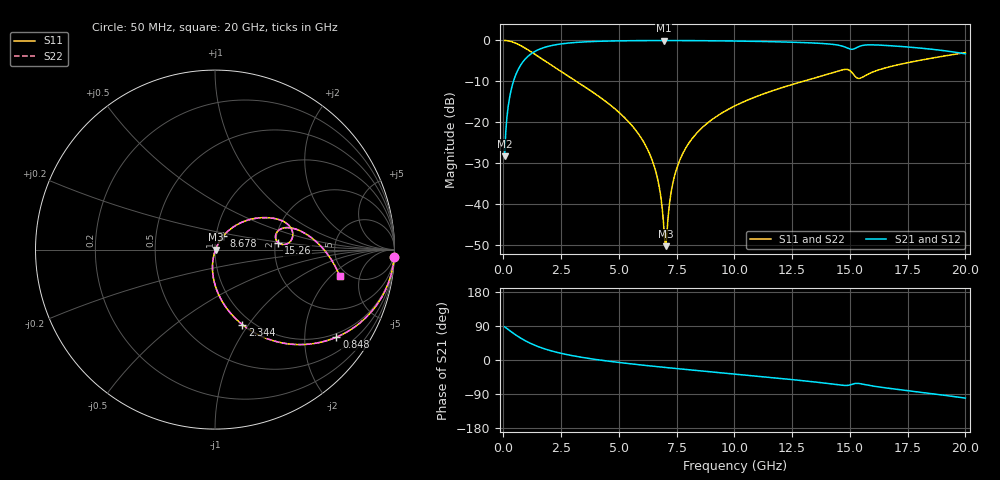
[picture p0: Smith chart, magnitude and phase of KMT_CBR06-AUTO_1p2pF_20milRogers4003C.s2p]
! Data measured by Modelithics Inc. support@modelithics.com 813-866-6335
! KEMET CBR06-AUTO 1.2pF, Pad Width= 0.851mm, Pad Length= 0.64mm, Pad Gap= 0.62mm, 20mil Rogers 4003C substrate Data, January 2022
# hz S ma R 50
! 2 Port Network Data from SP1.SP block
! freq  magS11  angS11  magS21  angS21  magS12  angS12  magS22  angS22
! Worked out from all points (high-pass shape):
!   401 points, 50 MHz to 20 GHz, reference 50 ohm
!   highest |S21| = -0.03 dB at 6.933 GHz (marker M1); lowest = -28.3 dB at 50 MHz (marker M2)
!   |S21| within 3 dB of the highest: 1.261 GHz to 19.73 GHz (18.47 GHz wide, 176 % of centre)
!   lowest |S11| = -50.3 dB at 7.032 GHz (marker M3), VSWR 1.01, Z = 50.3 - j0.0299 ohm
!   |S11| at or under -10 dB: 3.16 GHz to 12.96 GHz (9.804 GHz wide, 122 % of centre)
!   |S22| runs from -50.3 to 0.0 dB; largest |S21 - S12| = 0
!   S11 on the Smith chart (normalised r, x): 50 MHz: 1, -49; 848 MHz: 0.89, -2.84; 2.344 GHz: 0.90, -0.94; 8.678 GHz: 1.09, +0.17; 15.26 GHz: 2.08, +0.18; 20 GHz: 4.30, -2.57
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5e7  0.9993 -2.3  0.0384 87.7  0.0384 87.7  0.9993 -2.3
1.99625e8  0.9884 -9.3  0.1517 80.7  0.1517 80.7  0.9884 -9.3
3.4925e8  0.9655 -16.0  0.2597 73.9  0.2597 73.9  0.9655 -16.0
8.48e8  0.8339 -35.8  0.5508 54.1  0.5508 54.1  0.8339 -35.8
1.54625e9  0.6259 -55.5  0.7784 34.4  0.7784 34.4  0.6259 -55.5
2.34425e9  0.445 -70.0  0.8936 19.8  0.8936 19.8  0.445 -70.0
3.391625e9  0.2868 -82.5  0.9557 7.1  0.9557 7.1  0.2868 -82.5
5.73575e9  0.07942 -99.7  0.9939 -11.6  0.9939 -11.6  0.07942 -99.7
6.33425e9  0.04086 -101.5  0.9961 -15.5  0.9961 -15.5  0.04086 -101.5
6.73325e9  0.0169 -98.1  0.9967 -18.0  0.9967 -18.0  0.0169 -98.1
6.93275e9  0.005797 -78.6  0.9968 -19.2  0.9968 -19.2  0.005797 -78.6
7.0325e9  0.003068 -5.6  0.9968 -19.8  0.9968 -19.8  0.003068 -5.6
7.33175e9  0.01795 58.6  0.9965 -21.6  0.9965 -21.6  0.01795 58.6
7.581125e9  0.03164 61.3  0.9961 -23.1  0.9961 -23.1  0.03164 61.3
8.03e9  0.05584 61.0  0.995 -25.8  0.995 -25.8  0.05584 61.0
8.678375e9  0.08989 58.3  0.9923 -29.5  0.9923 -29.5  0.08989 58.3
1.0025e10  0.1589 51.4  0.9832 -37.2  0.9832 -37.2  0.1589 51.4
1.336662e10  0.3408 31.5  0.9319 -57.2  0.9319 -57.2  0.3408 31.5
1.4813e10  0.4429 13.3  0.8258 -67.2  0.8258 -67.2  0.4429 13.3
1.526188e10  0.3556 6.0  0.8087 -61.7  0.8087 -61.7  0.3556 6.0
1.670825e10  0.476 13.3  0.8632 -74.8  0.8632 -74.8  0.476 13.3
2e10  0.7102 -12.0  0.6857 -100.6  0.6857 -100.6  0.7102 -12.0
